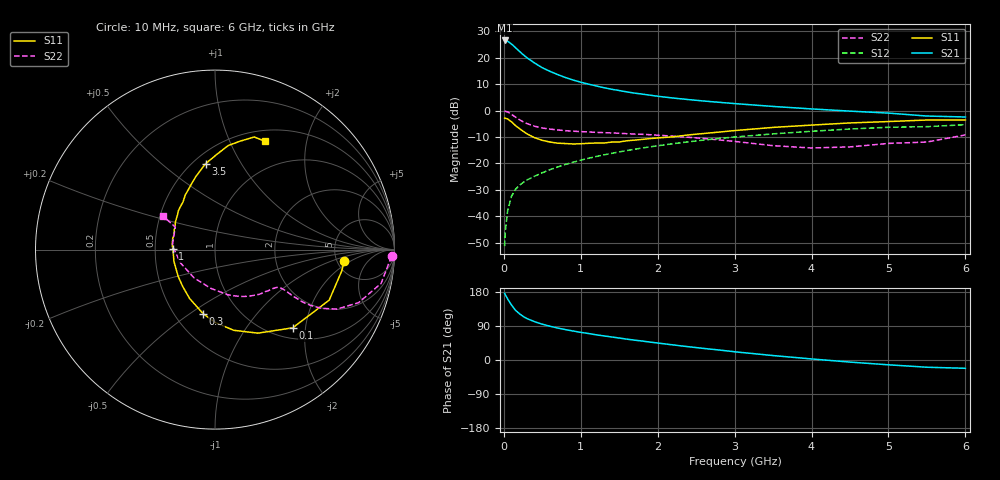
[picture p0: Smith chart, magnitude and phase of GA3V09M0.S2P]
! Infineon Technologies  Discrete & RF Semiconductors
! BF775
! Si NPN RF Bipolar Junction Transistor in SOT23
! VCE = 3 V  IC = 9 mA
! Common Emitter S-Parameters:  May  1996
# GHz  S  MA  R  50
!  f  S11  S21  S12  S22
! GHz  MAG  ANG  MAG  ANG  MAG  ANG  MAG  ANG
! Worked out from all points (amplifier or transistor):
!   36 points, 10 MHz to 6 GHz, reference 50 ohm
!   highest |S21| = 26.6 dB at 10 MHz (marker M1)
!   |S21| within 3 dB of that: start of sweep to 161.5 MHz
!   unconditionally stable (mu >= 1): 591.3 MHz to 3.328 GHz
!   at 250 MHz: K = 0.66, MSG = 24.2 dB, |S12| = -27.3 dB
!   at 1.4 GHz: K = 1.12, MAG = 10.0 dB, |S12| = -16.2 dB
!   at 6 GHz: K = 0.96, MSG = 1.5 dB, |S12| = -5.3 dB
!   S11 on the Smith chart (normalised r, x): 10 MHz: 5.83, -1.54; 100 MHz: 1.22, -1.70; 300 MHz: 0.69, -0.57; 1 GHz: 0.62, +0.01; 3.5 GHz: 0.57, +0.72; 6 GHz: 0.63, +1.36
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0.01  0.724 -5.0  21.39 176.0  0.0027 90.0  0.985 -2.2
0.02  0.7157 -9.7  21.34 171.9  0.0053 82.3  0.9707 -4.7
0.05  0.6957 -23.9  20.68 160.9  0.0129 78.2  0.9444 -11.5
0.1  0.6143 -45.2  18.28 145.0  0.0239 70.5  0.8529 -20.3
0.15  0.5234 -62.8  15.7 131.6  0.0321 64.5  0.756 -26.0
0.2  0.4616 -76.9  13.42 122.5  0.0382 62.1  0.6775 -28.9
0.25  0.4077 -89.4  11.54 115.1  0.0434 60.8  0.616 -30.3
0.3  0.3637 -100.4  10.09 109.3  0.0485 60.5  0.57 -30.9
0.4  0.3071 -117.4  7.979 101.1  0.0572 61.0  0.5068 -30.8
0.5  0.2735 -131.0  6.506 94.5  0.0664 61.8  0.4692 -30.4
0.6  0.2542 -143.6  5.548 89.1  0.0761 62.5  0.4469 -30.2
0.7  0.2417 -154.6  4.821 84.3  0.0854 63.2  0.4303 -30.2
0.8  0.2378 -164.3  4.246 80.2  0.0954 63.2  0.4175 -30.5
1  0.2357 178.9  3.458 73.0  0.1152 63.0  0.4009 -31.8
1.1  0.2404 172.0  3.179 69.9  0.1253 62.9  0.3945 -33.0
1.3  0.2427 160.5  2.723 63.6  0.1453 61.7  0.3828 -35.3
1.6  0.2688 145.3  2.265 55.0  0.1752 59.6  0.3655 -39.8
2.2  0.3188 124.1  1.734 39.8  0.2365 54.1  0.3286 -51.5
3.5  0.4814 96.3  1.201 11.7  0.3626 38.3  0.2168 -96.4
4.5  0.585 82.7  0.979 -5.5  0.4488 25.1  0.2056 -158.6
5.5  0.6644 70.8  0.79 -19.1  0.4973 10.4  0.2541 150.5
6  0.6647 65.3  0.758 -21.9  0.5412 6.3  0.3466 147.1
